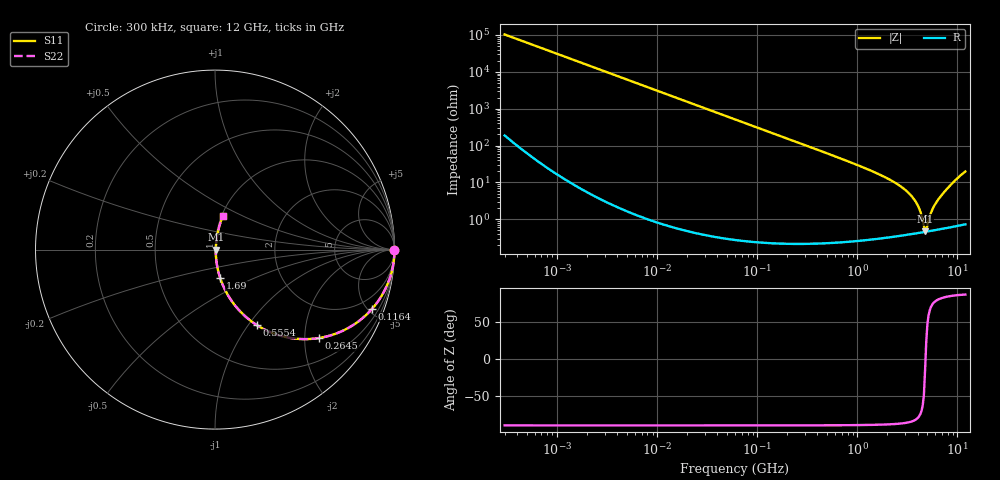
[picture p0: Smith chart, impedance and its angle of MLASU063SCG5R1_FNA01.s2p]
! MLASU063SCG5R1_FNA01  S-PARAMETER MODEL  ( Standard Model )
! Model Generated by TAIYO YUDEN Corporation (http://www.ty-top.com)
! Version 1.0
! TAIYO YUDEN Control No. 240819
! Copyright(c) 2024 TAIYO YUDEN CO.,LTD. All Rights Reserved.
! Product Description (link to TY-COMPAS)
! https://ds.yuden.co.jp/TYCOMPAS/or/detail?pn=MLASU063SCG5R1DFNA01&u=M
! Products Name : Multilayer Ceramic Capacitors
! Characteristics :
!  Capacitance : 5.1 [pF] , Rated Voltage : 50 [V] , TCC : CG / C0G
!  Case Size : 0.6 x 0.3 / 0.024 x 0.012 [mm/inch] , Thickness : 0.3 / 0.012 [mm/inch]
!  (Conditions: Temperature = 25 [degC] , DC Bias Voltage = 0 [V])
! External Node Assignments :
!  1  o---| |---o  2
! GND o---------o GND
! Frequency Range : 0.3MHz  -  12000MHz  [ 401 STEP ]
# MHZ S RI R 50
! Freq[MHz].  S11 Real  S11 Imag  S21 Real  S21 Imag  S12 Real  S12 Imag  S22 Real  S22 Imag
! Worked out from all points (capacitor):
!   401 points, 300 kHz to 12 GHz, reference 50 ohm
!   read as one part in series: C = 5.13 pF near 316.3 kHz
!   lowest |Z| = 471 mohm at 4.748 GHz (marker M1)
!   series resonance near 4.796 GHz, so ESL is about 210 pH
!   S11 on the Smith chart (normalised r, x): 300 kHz: open; 116.4 MHz: 1.00, -5.33; 264.5 MHz: 1.00, -2.34; 555.4 MHz: 1.00, -1.10; 1.69 GHz: 1.01, -0.32; 12 GHz: 1.01, +0.39
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0.3  1 -0.000967  2.7e-06 0.000967  2.7e-06 0.000967  1 -0.000967
1.769972  1 -0.0057  3.47e-05 0.0057  3.47e-05 0.0057  1 -0.0057
10.44266  0.9989 -0.0336  0.00114 0.0336  0.00114 0.0336  0.9989 -0.0336
27.82928  0.992 -0.089  0.00801 0.089  0.00801 0.089  0.992 -0.089
60  0.9638 -0.1864  0.0362 0.1864  0.0362 0.1864  0.9638 -0.1864
116.3536  0.8764 -0.3287  0.1236 0.3287  0.1236 0.3287  0.8764 -0.3287
264.5085  0.5775 -0.493  0.4225 0.493  0.4225 0.493  0.5775 -0.493
353.9943  0.4319 -0.4941  0.5681 0.4941  0.5681 0.4941  0.4319 -0.4941
555.3718  0.234 -0.4213  0.766 0.4213  0.766 0.4213  0.234 -0.4213
918.7169  0.0976 -0.2929  0.9024 0.2929  0.9024 0.2929  0.0976 -0.2929
1689.663  0.028 -0.156  0.972 0.156  0.972 0.156  0.028 -0.156
2088.533  0.0174 -0.118  0.9826 0.118  0.9826 0.118  0.0174 -0.118
2947.191  0.00793 -0.0649  0.9921 0.0649  0.9921 0.0649  0.00793 -0.0649
3642.919  0.00532 -0.0359  0.9947 0.0359  0.9947 0.0359  0.00532 -0.0359
4158.869  0.00462 -0.0186  0.9954 0.0186  0.9954 0.0186  0.00462 -0.0186
4623.766  0.0045 -0.00497  0.9955 0.00497  0.9955 0.00497  0.0045 -0.00497
4747.894  0.00453 -0.00119  0.9955 0.00119  0.9955 0.00119  0.00453 -0.00119
5006.236  0.00467 0.00507  0.9953 -0.00507  0.9953 -0.00507  0.00467 0.00507
5565.855  0.00516 0.0165  0.9948 -0.0165  0.9948 -0.0165  0.00516 0.0165
6524.734  0.00655 0.0356  0.9935 -0.0356  0.9935 -0.0356  0.00655 0.0356
9207.246  0.0169 0.1022  0.9831 -0.1022  0.9831 -0.1022  0.0169 0.1022
12000  0.044 0.1874  0.956 -0.1874  0.956 -0.1874  0.044 0.1874
